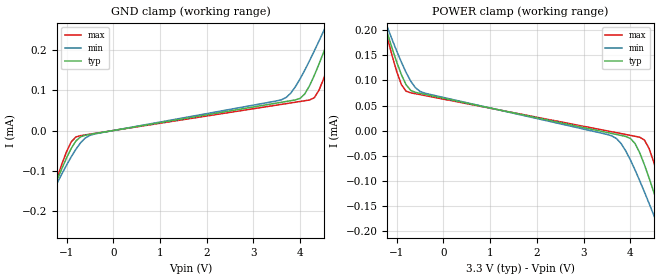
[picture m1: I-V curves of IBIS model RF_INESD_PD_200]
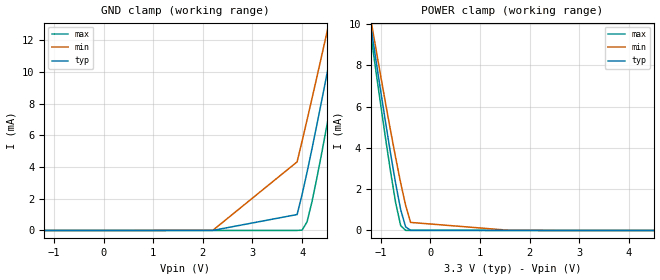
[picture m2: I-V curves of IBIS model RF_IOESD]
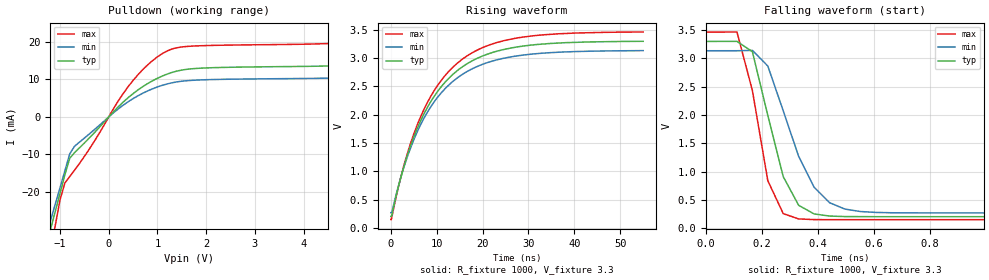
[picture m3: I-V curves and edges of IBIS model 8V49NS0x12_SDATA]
|   This file is an IBIS representation of the   |
|   Integrated Device Technology, Inc.   |
|   8T79S308   |
|   1:8 UNIVERSAL DIFFERENTIAL FANOUT BUFFER   |
[IBIS Ver]   4.1
[File name]   8t79s308.ibs
[Date]   16 Feb 2018
[Source]   Originated at Integrated Device Technology, Inc.
[Disclaimer]
IDT hereby grants the user of this IBIS model a non-exclusive,
nontransferable license to use this IBIS model under the following terms.
Before using this IBIS model, the user should read this license.
If the user does not accept these terms,  the IBIS model should be
returned to IDT within 30 days.
   The user is granted this license only to use the IBIS model and
is not granted rights to sell, load, rent, lease or license the IBIS
model in whole or in part, or in modified form to anyone other than
user. User may modify the IBIS model to suit its specific
applications but rights to derivative works and such modifications
shall belong to IDT.
   This IBIS model is provided on an "AS IS" basis and IDT makes
absolutely no warranty with respect to the information contained
herein. IDT DISCLAIMS AND CUSTOMER WAIVES ALL WARRANTIES, EXPRESS
OR IMPLIED, INCLUDING WARRANTIES OF MERCHANTABILITY OR FITNESS FOR
A PARTICULAR PURPOSE. The entire risk as to quality and performance
is with the Customer. ACCORDINGLY, IN NO EVENT SHALL THE COMPANY BE
LIABLE FOR ANY DAMAGES, WHETHER IN CONTRACT OR TORT,INCLUDING ANY
LOST PROFITS OR OTHER INCIDENTAL, CONSEQUENTIAL, EXEMPLARY, OR
PUNITIVE DAMAGES ARISING OUT OF THE USE OR APPLICATION OF THE IBIS
model provided in this package. Further, IDT reserves the right to
make changes without notice to any product herein to improve
reliability, function, or design. IDT does not convey any license
under patent rights or any other intellectual property rights,
including those of third parties.
   IDT is not obligated to provide maintenance or support
for the licensed IBIS model.
[Copyright] Copyright 2015 by Integrated Device Technology, Inc.
[Component]   8T79S308NLGI
[Manufacturer] Integrated Device Technology, Inc.
[Package]
|LD QFN 40
|lead + wire   typ   min   max
R_pkg   7.1539E-02   5.8459E-02   9.5092E-02
L_pkg   1.4325E-09   1.0877E-09   2.0537E-09
C_pkg   5.9801E-14   5.5325E-14   6.5653E-14
[Pin] signal_name  model_name   R_pin   L_pin   C_pin
1   PD_OE   RF_INESD_PD_200   8.5557E-02   1.8029E-09   6.3191E-14
2   VSEL_I2C   RF_INESD_PD_200   7.6183E-02   1.5542E-09   6.2015E-14
3   XSEL0   RF_INESD_PD_200   6.6383E-02   1.2964E-09   5.8526E-14
4   XSEL1   RF_INESD_PD_200   6.6920E-02   1.3109E-09   5.8763E-14
5   VDD   POWER   6.0741E-02   1.1478E-09   5.6176E-14
6   SCL   RF_IOESD   5.8459E-02   1.0877E-09   5.5325E-14
7   SDA   8V49NS0x12_SDATA   6.0207E-02   1.1343E-09   5.6120E-14
8   ADR0   RF_INESD_PD_200   6.3964E-02   1.2328E-09   5.7694E-14
9   ADR1   RF_INESD_PD_200   7.1615E-02   1.4340E-09   6.0514E-14
10  ARD2   RF_INESD_PD_200   8.6096E-02   1.8170E-09   6.3252E-14
11  VDDA   POWER   8.6631E-02   1.8312E-09   6.3484E-14
12  QA0   8T79S308_Qx   7.5512E-02   1.5366E-09   6.1638E-14
13  nQA0   8T79S308_Qx   6.6247E-02   1.2928E-09   5.8380E-14
14  QA1   8T79S308_Qx   6.0743E-02   1.1484E-09   5.6429E-14
15  nQA1   8T79S308_Qx   5.9668E-02   1.1195E-09   5.5855E-14
16  QA2   8T79S308_Qx   6.3966E-02   1.2326E-09   5.7537E-14
17  nQA2   8T79S308_Qx   7.3233E-02   1.4771E-09   6.1020E-14
18  QA3   8T79S308_Qx   8.2496E-02   1.7204E-09   6.3925E-14
19  nQA3   8T79S308_Qx   8.5045E-02   1.7874E-09   6.4649E-14
20  VDDA   POWER   9.5092E-02   2.0537E-09   6.5653E-14
21  VSEL_VDD   RF_INESD_PD_200   8.6362E-02   1.8241E-09   6.3205E-14
22  IN_0   RF_IOESD   7.0946E-02   1.4164E-09   6.0237E-14
23  nIN_0   RF_IOESD   6.8663E-02   1.3564E-09   5.9445E-14
24  VT_0   NC   6.5040E-02   1.2614E-09   5.8000E-14
25  VDD_IN_0   POWER   6.0742E-02   1.1479E-09   5.6257E-14
26  VDD_IN_1   POWER   6.1547E-02   1.1691E-09   5.6462E-14
27  VT_1   NC   6.4102E-02   1.2369E-09   5.7655E-14
28  nIN_1   RF_IOESD   6.7053E-02   1.3140E-09   5.8813E-14
29  IN_1   RF_IOESD   7.2958E-02   1.4693E-09   6.1096E-14
30  RES2   NC   8.6901E-02   1.8381E-09   6.3478E-14
31  VDDB   POWER   8.9987E-02   1.9196E-09   6.4336E-14
32  nQB3   8T79S308_Qx   8.0749E-02   1.6744E-09   6.3449E-14
33  QB3   8T79S308_Qx   6.9197E-02   1.3705E-09   5.9552E-14
34  nQB   8T79S308_Qx   7.0009E-02   1.3922E-09   6.0035E-14
35  QB2   8T79S308_Qx   6.1145E-02   1.1585E-09   5.6415E-14
36  nQB1   8T79S308_Qx   5.9937E-02   1.1266E-09   5.5909E-14
37  QB1   8T79S308_Qx   5.9804E-02   1.1237E-09   5.5979E-14
38  nQB0   8T79S308_Qx   6.5441E-02   1.2716E-09   5.8175E-14
39  QB0   8T79S308_Qx   7.3496E-02   1.4835E-09   6.1056E-14
40  VDDB   POWER   8.2738E-02   1.7286E-09   6.2354E-14
[Diff Pin]  inv_pin  vdiff tdelay_typ tdelay_min  tdelay_max
|Outputs
12   13   NA   0   0   0
14   15   NA   0   0   0
16   17   NA   0   0   0
18   19   NA   0   0   0
33   32   NA   0   0   0
35   34   NA   0   0   0
37   36   NA   0   0   0
39   38   NA   0   0   0
|Inputs
22   23   0.3   NA   NA   NA
29   28   0.3   NA   NA   NA
|Some simulators only recognize the 100ohm resistance across a differential
|pair.  This file is configured for such simulators.
|However, this configuration does not allow for the use of VT, pins 27 and 24, for biasing.
|The user can comment out the "Series Pin Mapping and "ODT_100" sections below
|and apply external components in order to use VT for biasing purposes.  In that
|case, for IN0 use a 50ohm resistor between pins 22 and 24 and another 50ohm resistor
|between pins 23 and 24. Do similar for IN1.
[Series Pin Mapping] Pin_2   model_name   function_table_group
22   23   ODT_100
28   28   ODT_100
[Model Selector] 8T79S308_Qx
LVPECL_750mV  3.3V LVPECL Driver, 750mV setting
LVDS_350mV   3.3V LVPECL Driver, 350mV setting
LVDS_500mV   3.3V LVPECL Driver, 500mV setting
[Model]   ODT_100
Model_type  Series
Polarity   Non-Inverting
|   typ   min   max
C_comp   0pF   0pF   0pF
|   typ   min   max
[Voltage Range]   3.3V   3.135V   3.465V
[R Series]   100ohm   90ohm   110ohm
| Models and submodels in the file (8): ODT_100 (Series), RF_INESD_PD_200 (Input), RF_IOESD (Input), 8V49NS0x12_SDATA (Open_drain), LVPECL_500mV (Output_ECL), LVPECL_750mV (Output_ECL), LVDS_500mV (Output), LVDS_350mV (Output)
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[Model]   RF_INESD_PD_200
Model_type   Input
Polarity   Non-Inverting
Vinl = 0.8V
Vinh = 2.0V
|   typ   min   max
C_comp   2pF   1.5pF   2.5pF
|   typ   min   max
[Voltage range]   3.3V   3.135V   3.465V
[GND_clamp]
|Voltage   I (typ)   I (min)   I (max)
|Note, modeling breaks down at 250mA and above.  This is well beyond the functional   |
|operating range of the device.  Should this scenario occur, catastrophic failure and   |
|possible damage to the device and/or board is of higher concern than the I-V curve   |
|behavior.  The IBIS checker will flag currents in excess of 10A with warnings.  Lines   |
|with currents in excess of 0.35 A have been commented out.  The points still remain|
|available to the user if the user desires to use them.   |
-3.3V     -781.2uA   -650.4uA   -919.6uA
-1.8V     -304.2uA   -274uA     -338.4uA
-1.6V     -242.4uA   -225.2uA   -262.9uA
-1V       -68.26uA   -86.19uA   -52.71uA
-800mV    -26.05uA   -46.59uA   -16uA
-400mV    -7.819uA   -8.648uA   -7.238uA
3.6V      70.37uA    76.64uA    65.15uA
4.2V      111.5uA    173.8uA    76.11uA
4.4V      164.8uA    222.4uA    99.75uA
4.7V      256.8uA    298.7uA    197.8uA
4.9V      321.2uA    350.9uA    273.2uA
6.6V      892.6uA    809.3uA    957uA
[Power_clamp]
|Voltage   I (typ)   I (min)   I (max)
|Note, modeling breaks down at 250mA and above.  This is well beyond the functional   |
|operating range of the device.  Should this scenario occur, catastrophic failure and   |
|possible damage to the device and/or board is of higher concern than the I-V curve   |
|behavior.  The IBIS checker will flag currents in excess of 10A with warnings.  Lines   |
|with currents in excess of 0.35 A have been commented out.  The points still remain|
|available to the user if the user desires to use them.   |
-3.3V     892.5uA    764.2uA    1.025mA
-1.3V     225.3uA    231.1uA    221.9uA
-1.2V     194.6uA    206.3uA    185.1uA
-900mV    111.5uA    136.5uA    91.79uA
-700mV    80.18uA    98.56uA    75.39uA
3.6V      -5.864uA   -10.63uA   -2.443uA
4.2V      -44.54uA   -100.3uA   -13.47uA
4.4V      -94.77uA   -145.6uA   -35.75uA
4.6V      -151.9uA   -192.7uA   -95.03uA
4.8V      -211.8uA   -241uA     -165uA
4.9V      -242.4uA   -265.4uA   -201.5uA
6.6V      -781.2uA   -692.4uA   -855uA
[Model]   RF_IOESD
Model_type   Input
Polarity   Non-Inverting
Vinl = 0.8V
Vinh = 2.0V
|   typ   min   max
C_comp   2pF   1.5pF   2.5pF
|   typ   min   max
[Voltage range]   3.3V   3.135V   3.465V
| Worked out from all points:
|   POWER clamp passes 1 mA (typ) near -0.60 V on its own axis
[GND_clamp]
|Voltage   I (typ)   I (min)   I (max)
-3.3V     -26.4pA    -29.17pA   -26.9pA
2.2V      3.884uA    6.52uA     2.085uA
3.9V      1.006mA    4.332mA    2.237uA
4V        2.26mA     5.637mA    20.46uA
4.1V      3.672mA    6.973mA    538uA
4.2V      5.164mA    8.333mA    1.82mA
4.5V      9.861mA    12.5mA     6.63mA
4.6V      11.47mA    13.9mA     8.341mA
4.7V      13.08mA    15.31mA    10.08mA
4.8V      14.7mA     16.73mA    11.83mA
4.9V      16.33mA    18.14mA    13.59mA
6.6V      43.33mA    41.8mA     43.26mA
[Power_clamp]
|Voltage   I (typ)   I (min)   I (max)
|Note, modeling breaks down at 250mA and above.  This is well beyond the functional   |
|operating range of the device.  Should this scenario occur, catastrophic failure and   |
|possible damage to the device and/or board is of higher concern than the I-V curve   |
|behavior.  The IBIS checker will flag currents in excess of 10A with warnings.  Lines   |
|with currents in excess of 0.35 A have been commented out.  The points still remain|
|available to the user if the user desires to use them.   |
-3.3V     43.35mA    39.59mA    45.99mA
-1.3V     11.47mA    11.59mA    11.21mA
-1.2V     9.862mA    10.19mA    9.466mA
-1.1V     8.272mA    8.812mA    7.739mA
-900mV    5.164mA    6.099mA    4.38mA
-800mV    3.672mA    4.782mA    2.791mA
-700mV    2.261mA    3.509mA    1.329mA
-600mV    1.006mA    2.301mA    234.8uA
-500mV    171.9uA    1.215mA    5.661uA
-400mV    10.05uA    390.1uA    2.096uA
1.6V      3.855uA    6.35uA     2.087uA
6.6V      -26.4pA    -29.99pA   -26.07pA
[Model]   8V49NS0x12_SDATA
Model_type   Open_drain
Polarity   Non-Inverting
|   typ   min   max
C_comp   2pF   1.5pF   2.5pF
Vmeas = 0.284V
Rref = 1000
Cref = 0
Vref = 1.65V
|   typ   min   max
[Voltage range]   3.3V   3.135V   3.465V
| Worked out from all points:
|   slope of the pulldown table from 0 to 0.495 V, typ, clamps not added: 80.5 ohm
|   rising waveform, R_fixture 1000, V_fixture 3.3: 20-80 % time 11.1ns typ, 11.1ns min, 11.1ns max; typ from 0.202 V to 3.3 V
|   falling waveform, R_fixture 1000, V_fixture 3.3: 20-80 % time 98.3ps typ, 132ps min, 77.2ps max; typ from 3.3 V to 0.202 V
[Pulldown]
|Voltage   I (typ)   I (min)   I (max)
|Note, modeling breaks down at 250mA and above.  This is well beyond the functional   |
|operating range of the device.  Should this scenario occur, catastrophic failure and   |
|possible damage to the device and/or board is of higher concern than the I-V curve   |
|behavior.  The IBIS checker will flag currents in excess of 10A with warnings.  Lines   |
|with currents in excess of 0.35 A have been commented out.  The points still remain|
|available to the user if the user desires to use them.   |
-3.3V     -130.8mA   -120.6mA   -175.6mA
-1.3V     -35.07mA   -32.27mA   -42.9mA
-1.2V     -30.19mA   -27.82mA   -36.01mA
-1.1V     -25.28mA   -23.34mA   -29.07mA
-900mV    -15.4mA    -14.33mA   -17.59mA
-800mV    -11mA      -9.8mA     -15.89mA
-700mV    -9.481mA   -7.782mA   -14.16mA
400mV     5.141mA    4.057mA    8.078mA
1.2V      11.41mA    8.788mA    17.58mA
1.9V      12.99mA    9.863mA    18.97mA
5.1V      13.85mA    10.56mA    20.03mA
6.6V      16.29mA    12.49mA    23.98mA
[Ramp]
|   typ   min   max
dV/dt_r   1.857/11.112n   1.718/11.113n   1.989/11.111n
dV/dt_f   1.859/0.098n   1.723/0.132n   1.99/0.077n
R_load =   50.0000
[Rising Waveform]
R_fixture = 1000
V_fixture = 3.3
V_fixture_min = 3.135
V_fixture_max = 3.465
C_fixture = 0.0p
| Time   typ   min   max
0s        202.3mV    269.1mV    149.7mV
220.2ps   226.2mV    272.4mV    188.2mV
1.762ns   762.4mV    772.7mV    759.7mV
3.303ns   1.205V     1.185V     1.232V
6.717ns   1.93V      1.859V     2.004V
10.79ns   2.475V     2.366V     2.585V
15.64ns   2.848V     2.714V     2.983V
21.25ns   3.075V     2.926V     3.226V
28.52ns   3.209V     3.05V      3.368V
55ns      3.297V     3.132V     3.461V
[Falling Waveform]
R_fixture = 1000
V_fixture = 3.3
V_fixture_min = 3.135
V_fixture_max = 3.465
C_fixture = 0.0p
| Time   typ   min   max
0s        3.3V       3.135V     3.465V
110.1ps   3.301V     3.135V     3.467V
165.2ps   3.118V     3.141V     2.432V
220.2ps   1.992V     2.865V     839.1mV
275.3ps   910.6mV    2.073V     256.5mV
330.3ps   403.6mV    1.269V     163mV
385.4ps   251.5mV    723mV      151mV
495.5ps   204.8mV    336.7mV    149.8mV
770.8ps   202.4mV    269.4mV    149.5mV
55ns      202.3mV    269.1mV    149.7mV
